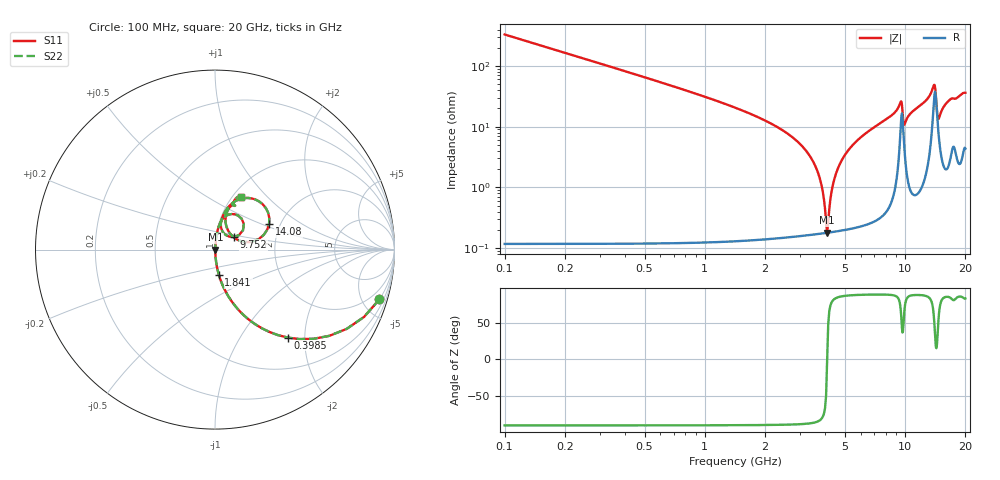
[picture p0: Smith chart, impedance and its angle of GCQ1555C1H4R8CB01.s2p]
!Murata Part Number: GCQ1555C1H4R8CB01
!These Parameters are Measured in Series Mode Connection
!Data Generated on Jan 08, 2026
!  o--ll--o
!Port1  Port2
!  o------o
!Operation Temp=25[degC], DC Bias Voltage=0[V]
!Freq. Start=100[MHz] Stop=20[GHz] 401[Steps]
# Hz S RI R 50
!Freq.(Hz) S11(Real) S11(Imag) S21(Real) S21(Imag) S12(Real) S12(Imag) S22(Real) S22(Imag)
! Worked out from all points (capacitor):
!   401 points, 100 MHz to 20 GHz, reference 50 ohm
!   read as one part in series: C = 4.8 pF near 199.5 MHz
!   lowest |Z| = 179 mohm at 4.08 GHz (marker M1)
!   series resonance near 4.082 GHz, so ESL is about 320 pH
!   S11 on the Smith chart (normalised r, x): 100 MHz: 1.00, -6.63; 398.5 MHz: 1.00, -1.65; 1.841 GHz: 1.00, -0.29; 9.752 GHz: 1.22, +0.17; 14.08 GHz: 1.75, +0.56; 20 GHz: 1.09, +0.72
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1e8  0.9165 -0.2765  0.0835 0.2765  0.0835 0.2765  0.9165 -0.2765
3.985e8  0.4046 -0.4901  0.5954 0.4901  0.5954 0.4901  0.4046 -0.4901
8.4625e8  0.1241 -0.3281  0.8759 0.3281  0.8759 0.3281  0.1241 -0.3281
1.84125e9  0.0215 -0.1404  0.9785 0.1404  0.9785 0.1404  0.0215 -0.1404
3.43325e9  0.00246 -0.0284  0.9975 0.0284  0.9975 0.0284  0.00246 -0.0284
3.7815e9  0.00188 -0.0125  0.9981 0.0125  0.9981 0.0125  0.00188 -0.0125
4.08e9  0.00178 -6.2e-05  0.9982 6.2e-05  0.9982 6.2e-05  0.00178 -6.2e-05
4.42825e9  0.00203 0.0134  0.998 -0.0134  0.998 -0.0134  0.00203 0.0134
4.82625e9  0.00271 0.0278  0.9973 -0.0278  0.9973 -0.0278  0.00271 0.0278
5.5725e9  0.00491 0.0526  0.9951 -0.0526  0.9951 -0.0526  0.00491 0.0526
6.7665e9  0.0106 0.0892  0.9894 -0.0892  0.9894 -0.0892  0.0106 0.0892
9.453e9  0.1087 0.197  0.8913 -0.197  0.8913 -0.197  0.1087 0.197
9.60225e9  0.1607 0.1432  0.8393 -0.1432  0.8393 -0.1432  0.1607 0.1432
9.7515e9  0.1061 0.0703  0.8939 -0.0703  0.8939 -0.0703  0.1061 0.0703
9.90075e9  0.0534 0.0873  0.9466 -0.0873  0.9466 -0.0873  0.0534 0.0873
1.005e10  0.0374 0.1109  0.9626 -0.1109  0.9626 -0.1109  0.0374 0.1109
1.338325e10  0.1376 0.2809  0.8624 -0.2809  0.8624 -0.2809  0.1376 0.2809
1.378125e10  0.2326 0.2757  0.7674 -0.2757  0.7674 -0.2757  0.2326 0.2757
1.407975e10  0.3013 0.1432  0.6987 -0.1432  0.6987 -0.1432  0.3013 0.1432
1.4627e10  0.0896 0.0825  0.9104 -0.0825  0.9104 -0.0825  0.0896 0.0825
1.67165e10  0.092 0.2446  0.908 -0.2446  0.908 -0.2446  0.092 0.2446
2e10  0.1439 0.2957  0.8561 -0.2957  0.8561 -0.2957  0.1439 0.2957
